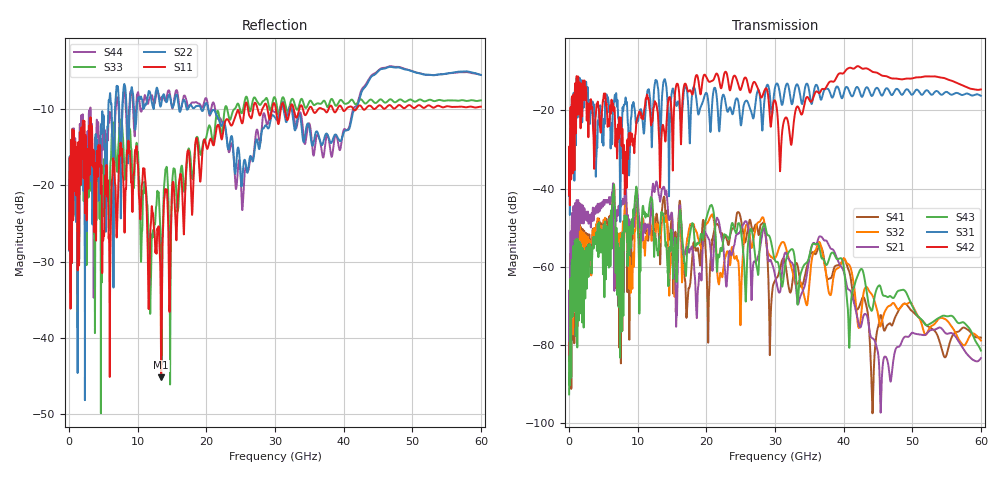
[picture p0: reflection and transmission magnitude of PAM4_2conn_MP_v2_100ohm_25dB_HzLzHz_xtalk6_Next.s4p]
! Info: Touchstone file created by Circ.  Input file=FAB50GbE_2conn_Midplane_Examax_Topo2_v2_100ohm_25dB_HzLzHz.circ
# Hz S RI R 50
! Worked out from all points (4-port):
!   6000 points, 10 MHz to 60 GHz, reference 50 ohm
!   strongest paths, dB at 10 MHz, 15.01 GHz, 30.01 GHz, 45.01 GHz, 60 GHz:
!     S42: -41.6, -24.7, -17.5, -10.5, -14.7
!     S31: -41.9, -15.0, -14.1, -14.4, -16.3
!     S43: -92.6, -52.4, -58.4, -65.0, -81.4
!     S21: -78.8, -46.6, -62.2, -82.0, -83.4
!     S32: -78.4, -53.7, -57.8, -72.1, -78.8
!     S41: -84.1, -47.5, -63.6, -75.4, -78.1
!   lowest |S11| = -45.2 dB at 13.42 GHz (marker M1), VSWR 1.01, Z = 50.5 + j0.153 ohm
!   |S11| at or under -10 dB: start of sweep to 25.58 GHz; 35.43 GHz to 36.33 GHz (893.9 MHz wide, 2.49 % of centre); 36.89 GHz to 37.81 GHz (922.4 MHz wide, 2.47 % of centre)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
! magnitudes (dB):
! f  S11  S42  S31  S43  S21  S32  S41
! 10 MHz  -28.4  -41.6  -41.9  -92.6  -78.8  -78.4  -84.1
! 1.34 GHz  -14.7  -11.6  -11.4  -55.4  -43.0  -50.5  -49.8
! 13.42 GHz  -45.2  -28.9  -22.6  -46.3  -41.5  -51.0  -49.4
! 15.51 GHz  -24.5  -14.6  -17.9  -53.4  -65.4  -60.4  -51.3
! 25.72 GHz  -9.3  -11.6  -17.6  -68.6  -48.3  -49.7  -53.4
! 30.8 GHz  -10.3  -33.6  -16.7  -62.7  -66.0  -54.3  -60.1
! 60 GHz  -9.7  -14.7  -16.3  -81.4  -83.4  -78.8  -78.1
